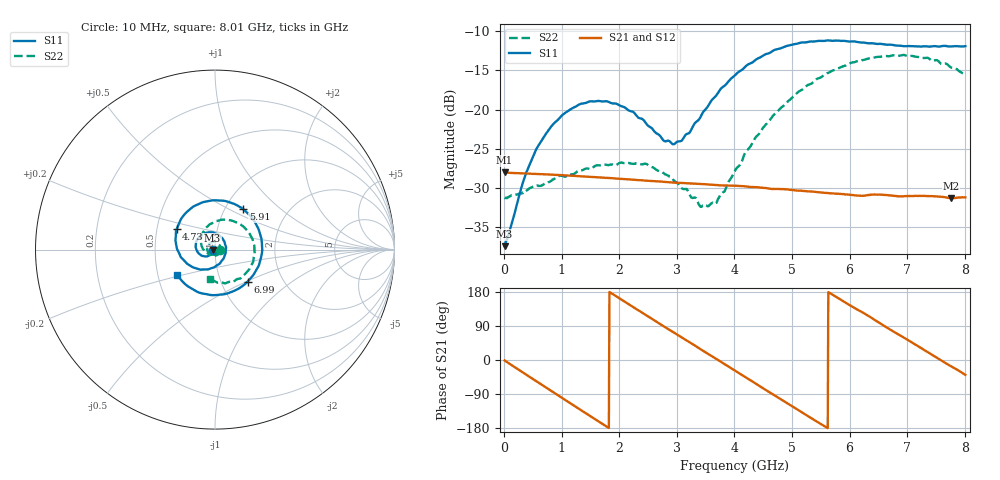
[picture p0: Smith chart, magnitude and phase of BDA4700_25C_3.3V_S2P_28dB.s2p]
!Agilent Technologies,E5071B,MY42404982,A.09.10
!Date: Mon Oct 20 18:14:50 2025
!Data & Calibration Information:
!Freq	S11:SOLT2(ON)	S21:SOLT2(ON)	S12:SOLT2(ON)	S22:SOLT2(ON)
# Hz S RI R 50
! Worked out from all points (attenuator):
!   801 points, 10 MHz to 8.01 GHz, reference 50 ohm
!   highest |S21| = -28.05 dB at 10 MHz (marker M1); lowest = -31.3 dB at 7.76 GHz (marker M2)
!   lowest |S11| = -37.5 dB at 10 MHz (marker M3), VSWR 1.03, Z = 48.7 - j0.138 ohm
!   |S11| at or under -10 dB: start of sweep to end of sweep
!   |S22| runs from -32.5 to -13.0 dB; largest |S21 - S12| = 0.00041
!   S11 on the Smith chart (normalised r, x): 10 MHz: 0.97, -0.00; 4.73 GHz: 0.63, +0.15; 5.91 GHz: 1.21, +0.59; 6.99 GHz: 1.33, -0.51; 8.01 GHz: 0.63, -0.19
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1e7  -0.0133 -0.00141  0.0396 -0.000841  0.0396 -0.000848  0.0272 -0.000821
3.5e8  -0.0244 -0.0267  0.0319 -0.0225  0.0318 -0.0224  0.0229 -0.0185
5.8e8  -0.0436 -0.0375  0.0205 -0.0328  0.0205 -0.0328  0.0145 -0.0292
1e9  -0.088 -0.0239  -0.00615 -0.0375  -0.00613 -0.0375  -0.0146 -0.0348
1.35e9  -0.1079 0.0169  -0.0258 -0.027  -0.0258 -0.027  -0.0365 -0.0183
1.97e9  -0.0566 0.0921  -0.035 0.00875  -0.0351 0.00872  -0.0349 0.0278
2.68e9  0.0516 0.0463  -0.00475 0.0344  -0.00474 0.0343  0.0128 0.0384
2.93e9  0.0599 -0.00169  0.00932 0.0328  0.00932 0.0327  0.025 0.0256
3.06e9  0.0559 -0.0283  0.0161 0.0299  0.0158 0.03  0.0278 0.0157
3.44e9  0.00228 -0.094  0.03 0.0146  0.03 0.0146  0.0199 -0.0136
3.69e9  -0.0565 -0.1102  0.0328 0.00132  0.0329 0.00124  0.00167 -0.0253
4.01e9  -0.14 -0.0884  0.0287 -0.0153  0.0287 -0.0153  -0.031 -0.026
4.39e9  -0.2106 0.00139  0.0138 -0.0287  0.0139 -0.0287  -0.0676 0.00371
4.73e9  -0.2142 0.1132  -0.00349 -0.0308  -0.00327 -0.0308  -0.0789 0.0538
5.35e9  -0.0559 0.2666  -0.0271 -0.0126  -0.027 -0.0128  -0.0158 0.1469
5.91e9  0.1572 0.2255  -0.0257 0.013  -0.0256 0.0128  0.109 0.1559
6.29e9  0.2469 0.1  -0.0141 0.0244  -0.0137 0.0245  0.1862 0.0977
6.68e9  0.2514 -0.0649  0.00363 0.028  0.00366 0.0281  0.2192 0.000456
6.99e9  0.1811 -0.1784  0.0161 0.0228  0.0162 0.0228  0.2052 -0.0819
7.39e9  0.0243 -0.2512  0.0266 0.00841  0.0266 0.00837  0.1341 -0.1624
7.76e9  -0.1353 -0.2142  0.026 -0.00772  0.026 -0.00778  0.0323 -0.1828
8.01e9  -0.2132 -0.1389  0.0212 -0.0173  0.0213 -0.0173  -0.0298 -0.1638
